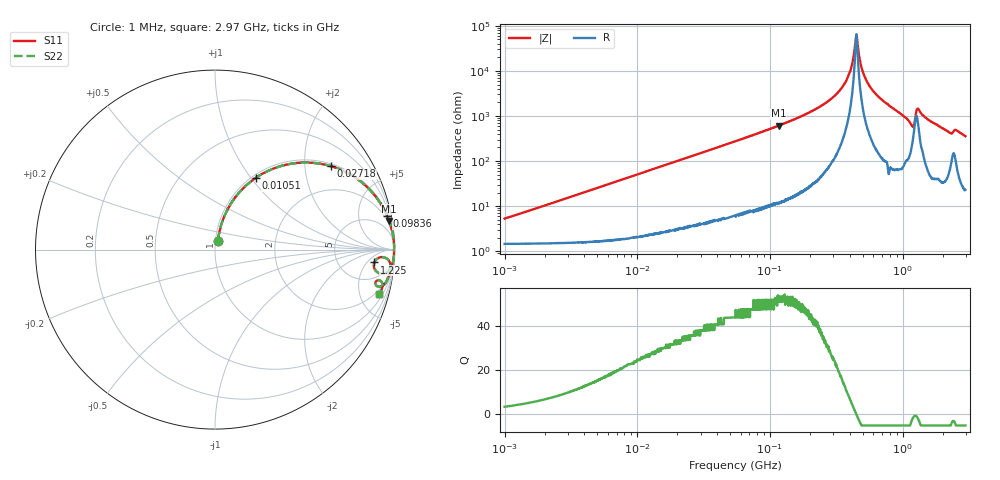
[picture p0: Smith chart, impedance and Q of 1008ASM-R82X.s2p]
!s-Parameter Generated by FASTRON Sdn. Bhd.
!FASTRON P/N : 1008ASM-R82X
!Keysight Technologies: E4991B_MY54100416_A.01.15
!Date: Tue Nov 21 09:36:05 2023
!Version  :Rev00  Wed Nov 22 15:17:41 2023
!Data & Calibration Information:
!Freq  S11  S21  S12  S22
!PortZ  Port1:50+j0  Port2:50+j0
!When reading reference impedance value at option line is always used.
! Remarks : This data is being provided solely for informational purposes.
# Hz S dB R 50
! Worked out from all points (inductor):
!   1599 points, 1 MHz to 2.97 GHz, reference 50 ohm
!   read as one part in series: L = 809 nH near 1.036 MHz
!   highest Q = 52.1 at 116 MHz (marker M1), where L = 832 nH
!   self-resonance near 448 MHz
!   S11 on the Smith chart (normalised r, x): 1 MHz: 1.03, +0.10; 10.51 MHz: 1.04, +1.06; 27.18 MHz: 1.07, +2.72; 98.36 MHz: 1, +10; 1.225 GHz: 12, -8; 2.97 GHz: 1.46, -7.15
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1000000  -25.70 71.2  -0.14 -2.9  -0.14 -2.9  -25.70 71.2
3804036  -14.60 74.6  -0.29 -10.7  -0.29 -10.7  -14.60 74.6
1.05052e7  -6.73 60.3  -1.21 -27.4  -1.21 -27.4  -6.73 60.3
1.439846e7  -4.77 52.8  -1.97 -35.2  -1.97 -35.2  -4.77 52.8
2.718395e7  -1.99 35.8  -4.66 -52.7  -4.66 -52.7  -1.99 35.8
5.477226e7  -0.60 19.8  -9.38 -68.9  -9.38 -68.9  -0.60 19.8
9.836149e7  -0.20 11.1  -14.30 -77.8  -14.30 -77.8  -0.20 11.1
1.160221e8  -0.14 9.3  -15.80 -79.6  -15.80 -79.6  -0.14 9.3
2.073156e8  -0.04 4.4  -22.20 -84.2  -22.20 -84.2  -0.04 4.4
2.884452e8  -0.02 2.4  -27.60 -85.5  -27.60 -85.5  -0.02 2.4
3.576934e8  -0.01 1.2  -33.60 -84.7  -33.60 -84.7  -0.01 1.2
4.033367e8  -0.01 0.6  -40.10 -80.8  -40.10 -80.8  -0.01 0.6
4.480278e8  -0.01 0.0  -56.20 -0.7  -56.20 -0.7  -0.01 0.0
4.593788e8  -0.01 -0.1  -51.20 55.5  -51.20 55.5  -0.01 -0.1
4.902556e8  -0.01 -0.5  -41.40 78.5  -41.40 78.5  -0.01 -0.5
5.337858e8  -0.02 -0.9  -35.70 83.2  -35.70 83.2  -0.02 -0.9
7.846996e8  -0.03 -3.3  -24.80 85.0  -24.80 85.0  -0.03 -3.3
1.171007e9  -0.55 -8.2  -16.30 62.1  -16.30 62.1  -0.55 -8.2
1.22495e9  -1.01 -4.6  -17.50 32.5  -17.50 32.5  -1.01 -4.6
1.313842e9  -0.27 -3.6  -23.30 62.1  -23.30 62.1  -0.27 -3.6
2.020405e9  -0.26 -10.6  -14.70 75.7  -14.70 75.7  -0.26 -10.6
2.970126e9  -0.47 -15.3  -11.50 71.0  -11.50 71.0  -0.47 -15.3
